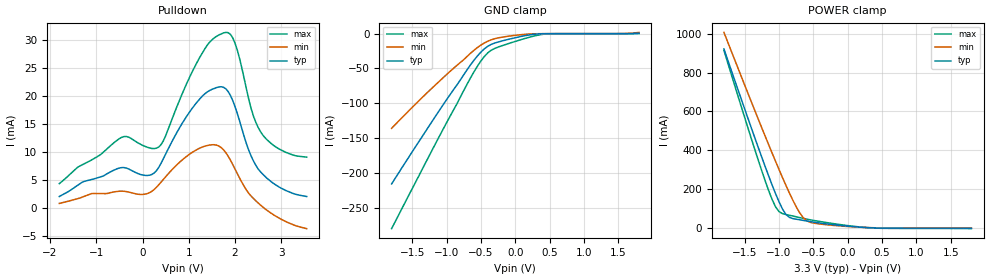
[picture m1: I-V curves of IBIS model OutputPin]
[IBIS Ver]   2.1
[File Name]   bug31.ibs
[File Rev]   0.1
[Component]   TEST
[Manufacturer]   Test File
[Package]
| variable   typ   min   max
R_pkg   0.0m   NA   NA
L_pkg   0.0nH   NA   NA
C_pkg   0.0pF   NA   NA
[Pin]   signal_name   model_name
1   One_Pin   OutputPin
| Models and submodels in the file (1): OutputPin (Output)
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[Model]   OutputPin
Model_type   Output
Vmeas = 1.2V
Cref = 5pF
Rref = 50
Vref = 1.2
| variable   typ   min   max
C_comp   6.763pF   NA   NA
[Temperature Range]   25.0   NA   NA
[Voltage range]   3.3V   NA   NA
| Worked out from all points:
|   slope of the pulldown table from 0 to 0.495 V, typ, clamps not added: 135 ohm
[Pulldown]
|   Voltage   I(typ)   I(min)   I(max)
-1.8V     2.092mA    849.8uA    4.399mA
-450mV    7.255mA    3.047mA    12.66mA
100mV     5.85mA     2.606mA    10.9mA
350mV     7.282mA    4.178mA    10.94mA
1.25V     19.65mA    10.78mA    27.13mA
1.6V      21.55mA    11.28mA    30.71mA
1.8V      21.35mA    9.937mA    31.42mA
2V        18.16mA    NA         29.49mA
2.35V     9.285mA    2.155mA    17.76mA
2.55V     6.516mA    NA         13.69mA
2.95V     3.8mA      NA         10.59mA
3.55V     2.09mA     -3.655mA   9.119mA
[GND Clamp]
|   Voltage   I(typ)   I(min)   I(max)
-1.8V     -216mA     -136.2mA   -280.3mA
-1.25V    -132.1mA   -81.88mA   -175mA
-700mV    -51.68mA   -32.66mA   -72.36mA
-550mV    -31.98mA   -19.95mA   -46.63mA
-450mV    -21.85mA   -13.43mA   -32.79mA
-400mV    -18.17mA   -10.9mA    -27.62mA
-300mV    -13.6mA    -7.369mA   -21.31mA
-200mV    -10.77mA   -5.282mA   -17.64mA
150mV     -2.827mA   -961.6uA   -6.751mA
400mV     -213.1uA   -102.5uA   -1.039mA
1.55V     -71.81uA   52.94uA    -75uA
1.8V      576.6uA    1.719mA    12.63uA
[POWER Clamp]
|   Voltage   I(typ)   I(min)   I(max)
-1.8V     922.2mA    1.008A     914.8mA
-1.3V     413.7mA    560.1mA    348.1mA
-1.15V    268.3mA    429.3mA    192.7mA
-1.05V    177.2mA    343.9mA    109mA
-1V       135.4mA    302mA      84.31mA
-900mV    70.21mA    220.6mA    68.71mA
-850mV    54.52mA    181.6mA    64.94mA
-700mV    41.94mA    78.73mA    53.07mA
-600mV    35.54mA    37.52mA    45.46mA
-350mV    22.38mA    17.61mA    29.71mA
350mV     113.8uA    887uA      -351.8uA
1.8V      -2.217mA   -1.009mA   -4.12mA
[Ramp]
|   typ   min   max
dV/dt_r   1.0/1.0n   NA   NA
dV/dt_f   1.0/1.0n   NA   NA
